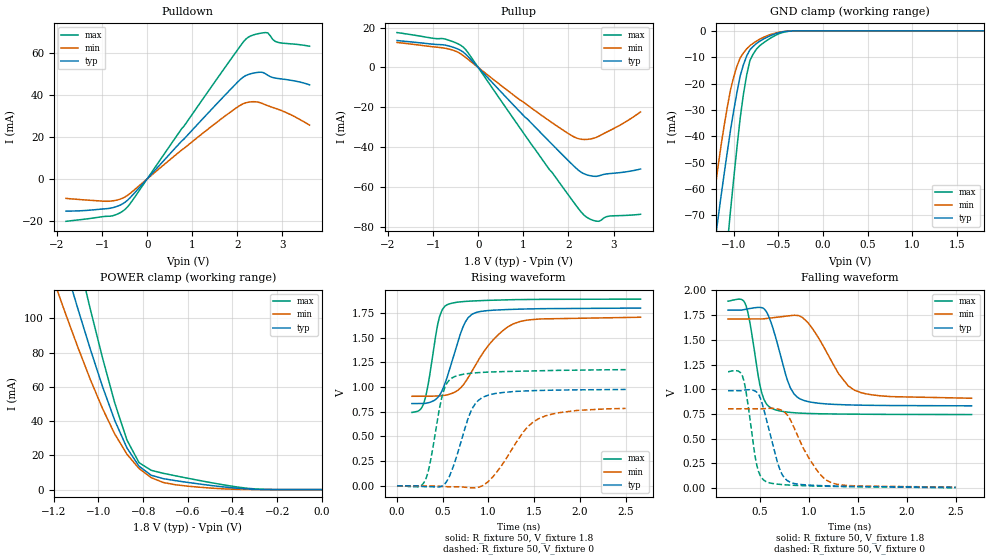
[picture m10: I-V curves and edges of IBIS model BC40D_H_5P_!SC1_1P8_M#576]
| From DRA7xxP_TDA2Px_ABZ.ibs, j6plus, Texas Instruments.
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| Model based on original model for BC1833DV40DCPBFBP1811_SSCEH
|   Sub model BC40D_H_5P_!SC1_1P8
[model]   BC40D_H_5P_!SC1_1P8_M#576
|[Description]  [1.8V-I/O-X-40D CLASS MODE FAST MODE, IND, 5 PERCENT%]
|   40D CLASS MODE FAST MODE, ,IND,5 PERCENT%
|[Input Load]
|[Output Drive] 40D CLASS MODE FAST MODE
|Voltage   1.8V
|Mode   I/O
Model_type   I/O
Polarity   Non-Inverting
Enable   Active-Low
Vinl =  0.63
Vinh =  1.17
Cref =  15pF
Rref =  100.0000M
Vref =  0V
Vmeas =  0.9
C_comp   2.29p   1.81p   2.77p
[Model Spec]
Vinl   0.63   0.5985   0.6615
Vinh   1.17   1.1115   1.2285
D_overshoot_ampl_h 0.36 0.36 0.36
D_overshoot_ampl_l 0.36 0.36 0.36
D_overshoot_area_h 0.33n 0.33n 0.33n
D_overshoot_area_l 0.33n 0.33n 0.33n
D_overshoot_high 2.16 2.16 2.16
D_overshoot_low -0.36 -0.36 -0.36
D_overshoot_time 1n 1n 1n
S_overshoot_high 1.8 1.8 1.8
S_overshoot_low 0 0 0
[Temperature Range]   25   125   -40
[Voltage Range]   1.8   1.71   1.89
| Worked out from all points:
|   slope of the pulldown table from 0 to 0.27 V, typ, clamps not added: 42.1 ohm
|   slope of the pullup table from 0 to 0.27 V, typ, clamps not added: 41.1 ohm
|   GND clamp passes 1 mA (typ) near -0.52 V on its own axis
|   POWER clamp passes 1 mA (typ) near -0.39 V on its own axis
|   rising waveform, R_fixture 50, V_fixture 1.8: 20-80 % time 200ps typ, 370ps min, 122ps max; typ from 0.832 V to 1.8 V
|   rising waveform, R_fixture 50, V_fixture 0: 20-80 % time 207ps typ, 359ps min, 141ps max; typ from -0.001 V to 0.975 V
|   falling waveform, R_fixture 50, V_fixture 1.8: 20-80 % time 170ps typ, 295ps min, 116ps max; typ from 1.8 V to 0.833 V
|   falling waveform, R_fixture 50, V_fixture 0: 20-80 % time 157ps typ, 258ps min, 104ps max; typ from 0.986 V to 0.009 V
[POWER_clamp]
-1.8V     435.3mA    358.7mA    550.4mA
-1.182V   145.1mA    115.2mA    186mA
-1.164V   136.9mA    108.6mA    175.7mA
-1.109V   112.9mA    89.05mA    145.1mA
-1.055V   89.59mA    70.36mA    115.1mA
-927.3mV  40.44mA    32.49mA    50.68mA
-872.7mV  24.38mA    20.7mA     29mA
-818.2mV  13.61mA    12.29mA    15.69mA
-763.6mV  8.369mA    6.958mA    11.24mA
-654.5mV  5.219mA    2.811mA    8.041mA
-327.3mV  349.6uA    49.46uA    691.6uA
0V        2.268uA    902.8nA    4.994uA
[Pulldown]
-1.8V     -15.33mA   -9.29mA    -20.21mA
-763.6mV  -13.73mA   -10.46mA   -17.56mA
-600mV    -12.51mA   -9.657mA   -16.14mA
-436.4mV  -10.18mA   -7.846mA   -13.35mA
1.473V    34.18mA    25.79mA    45.39mA
2.073V    47.54mA    35.19mA    63.55mA
2.236V    49.7mA     36.52mA    67.45mA
2.509V    50.84mA    36.26mA    69.39mA
2.673V    49.38mA    34.87mA    69.6mA
2.782V    48.33mA    34.06mA    66.49mA
2.891V    47.87mA    33.25mA    65.1mA
3.6V      44.82mA    25.63mA    63.22mA
[Pullup]
-1.8V     13.52mA    12.56mA    17.53mA
-763.6mV  11.34mA    9.77mA     14.43mA
-490.9mV  9.653mA    8.093mA    12.32mA
-327.3mV  7.63mA     5.886mA    10.14mA
-218.2mV  5.3mA      3.95mA     7.201mA
927.3mV   -22.34mA   -16.33mA   -30.45mA
1.909V    -44.8mA    -31.9mA    -61.25mA
2.236V    -51.88mA   -35.87mA   -71.32mA
2.4V      -53.89mA   -36.17mA   -75.15mA
2.618V    -54.71mA   -35.13mA   -77.23mA
2.891V    -53.38mA   -31.97mA   -74.74mA
3.6V      -51.01mA   -22.34mA   -73.77mA
[GND_clamp]
-1.8V     -241.7mA   -231.6mA   -367.4mA
-1.255V   -91.62mA   -71.7mA    -149.9mA
-1.182V   -72.85mA   -53.19mA   -122mA
-1.073V   -46.19mA   -29.16mA   -81.51mA
-1.036V   -37.83mA   -22.49mA   -68.45mA
-927.3mV  -17.13mA   -10.25mA   -33.06mA
-890.9mV  -12.84mA   -8.372mA   -24.01mA
-818.2mV  -7.187mA   -5.618mA   -11.22mA
-745.5mV  -4.828mA   -3.893mA   -6.943mA
-563.6mV  -1.493mA   -1.147mA   -2.288mA
-381.8mV  -98.54uA   -88.42uA   -167.6uA
1.8V      2.268uA    1.016uA    4.793uA
[Ramp]
dV/dt_f   0.598188/0.17546631n   0.50631/0.31108391n   0.700584/0.11831175n
dV/dt_r  0.5998134/0.21387135n   0.494352/0.38433897n  0.7131996/0.14280807n
R_load = 50
[Rising Waveform]
R_fixture = 50
V_fixture = 1.8
V_fixture_min = 1.71
V_fixture_max = 1.89
163.3ps   831.9mV    905.5mV    742.3mV
295.8ps   832.4mV    905.5mV    843.7mV
341.6ps   839.8mV    906.3mV    1.032V
446ps     893.3mV    909.7mV    1.638V
546.1ps   1.093V     919.5mV    1.832V
711.9ps   1.586V     1.007V     1.864V
849.7ps   1.749V     1.209V     1.872V
1.097ns   1.78V      1.519V     1.88V
1.349ns   1.788V     1.664V     1.885V
2.663ns   1.799V     1.706V     1.889V
[Rising Waveform]
R_fixture = 50
V_fixture = 0
V_fixture_min = 0
V_fixture_max = 0
0s        -789.9uV   -804.8uV   -729.9uV
303.3ps   -10.15mV   -1.901mV   45.7mV
356ps     -10.4mV    -2.523mV   204.6mV
489.8ps   -4.627mV   -7.727mV   897.3mV
544.3ps   44.98mV    -10.22mV   1.037V
620.5ps   208mV      -10.56mV   1.101V
802.9ps   742.7mV    -20.88mV   1.138V
951.2ps   900.7mV    9.623mV    1.148V
1.545ns   964.3mV    676.6mV    1.163V
2.5ns     974.5mV    782.5mV    1.175V
[Falling Waveform]
R_fixture = 50
V_fixture = 1.8
V_fixture_min = 1.71
V_fixture_max = 1.89
172.3ps   1.8V       1.71V      1.891V
355.9ps   1.81V      1.71V      1.848V
517ps     1.825V     1.71V      963.4mV
623.1ps   1.644V     1.722V     805.1mV
810.6ps   1.013V     1.744V     765.6mV
926.3ps   894.7mV    1.73V      758mV
1.057ns   864.1mV    1.584V     753.8mV
1.303ns   845.2mV    1.158V     749.7mV
1.468ns   840.2mV    990mV      748.1mV
2.663ns   832.6mV    909.4mV    744.4mV
[Falling Waveform]
R_fixture = 50
V_fixture = 0
V_fixture_min = 0
V_fixture_max = 0
172.3ps   985.8mV    802.4mV    1.178V
321.4ps   988.1mV    802.4mV    1.13V
356.1ps   993.6mV    802.4mV    979.5mV
467.9ps   968.9mV    802.4mV    227.4mV
559.7ps   714.6mV    805.8mV    66.95mV
704ps     185mV      794.1mV    38.32mV
811.1ps   58.88mV    688.4mV    30.89mV
1.051ns   28.73mV    226.1mV    21.57mV
1.235ns   22.41mV    53.1mV     18.27mV
2.5ns     9.378mV    10.7mV     3.421mV
